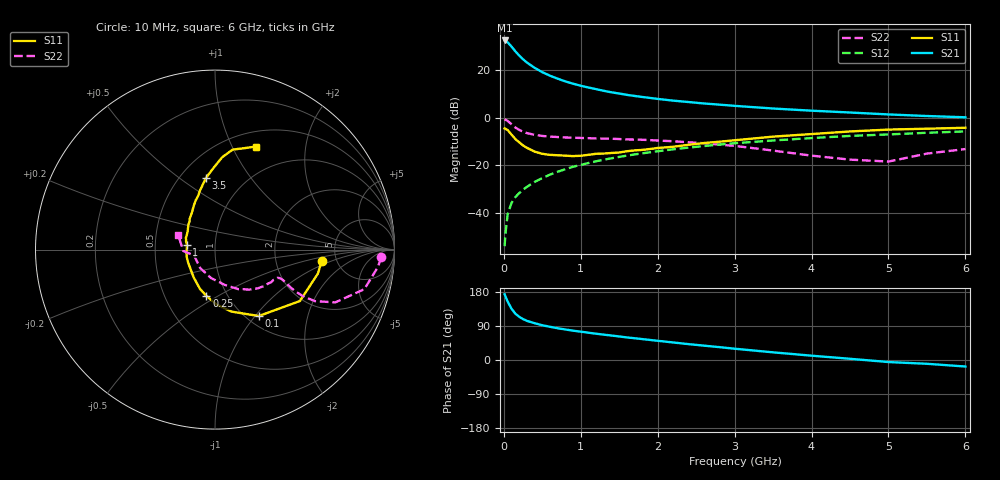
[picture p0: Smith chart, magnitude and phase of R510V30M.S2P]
! SIEMENS Small Signal Semiconductors
! BFR183
! Si NPN RF Bipolar Junction Transistor in SOT23
! VCE = 10 V  IC = 30 mA
! Common Emitter S-Parameters:  May  1996
# GHz  S  MA  R  50
!  f  S11  S21  S12  S22
! GHz  MAG  ANG  MAG  ANG  MAG  ANG  MAG  ANG
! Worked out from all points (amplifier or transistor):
!   36 points, 10 MHz to 6 GHz, reference 50 ohm
!   highest |S21| = 32.5 dB at 10 MHz (marker M1)
!   |S21| within 3 dB of that: start of sweep to 110.2 MHz
!   unconditionally stable (mu >= 1): 517 MHz to 2.553 GHz
!   at 250 MHz: K = 0.84, MSG = 27.4 dB, |S12| = -30.2 dB
!   at 1.4 GHz: K = 1.04, MAG = 12.6 dB, |S12| = -17.0 dB
!   at 6 GHz: K = 0.90, MSG = 3.0 dB, |S12| = -5.7 dB
!   S11 on the Smith chart (normalised r, x): 10 MHz: 3.80, -0.78; 100 MHz: 1.13, -1.04; 250 MHz: 0.80, -0.44; 1 GHz: 0.73, +0.04; 3.5 GHz: 0.66, +0.63; 6 GHz: 0.67, +1.24
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0.01  0.5977 -6.3  42.35 173.5  0.002 71.9  0.9278 -2.6
0.02  0.5887 -13.1  41.73 168.2  0.0035 79.3  0.9128 -6.1
0.05  0.5531 -31.2  38.66 154.0  0.0094 74.8  0.8612 -14.8
0.1  0.4432 -56.6  31.42 135.3  0.0163 69.5  0.7317 -23.7
0.15  0.3575 -75.1  24.99 122.2  0.0216 68.5  0.6257 -27.3
0.2  0.3053 -88.7  20.4 114.1  0.0261 69.3  0.5562 -27.9
0.25  0.262 -100.6  17.01 107.9  0.0309 69.6  0.5091 -27.5
0.3  0.2337 -111.2  14.55 103.3  0.0353 69.9  0.4771 -26.8
0.4  0.1945 -127.9  11.26 97.1  0.0449 71.5  0.4387 -25.2
0.5  0.1749 -140.8  9.117 91.7  0.0541 72.1  0.4157 -24.2
0.6  0.1664 -154.1  7.68 87.6  0.0639 72.2  0.4032 -23.8
0.7  0.1632 -164.3  6.649 83.8  0.0734 72.3  0.3941 -23.8
0.8  0.1602 -174.1  5.829 80.5  0.0831 71.2  0.3862 -24.1
1  0.1592 169.9  4.729 74.7  0.1022 70.2  0.3772 -25.2
1.1  0.1671 164.6  4.337 72.1  0.1121 69.5  0.3732 -26.5
1.3  0.1773 152.2  3.694 66.9  0.132 67.8  0.3649 -28.3
1.6  0.1985 138.7  3.039 59.6  0.1604 64.8  0.3515 -32.4
2.2  0.2458 121.2  2.3 46.3  0.2176 58.1  0.322 -42.1
3.5  0.4021 97.2  1.569 20.2  0.3338 41.8  0.2045 -74.4
4.5  0.5167 85.5  1.293 3.2  0.4166 29.4  0.132 -128.7
5.5  0.5905 73.4  1.091 -10.0  0.4848 18.3  0.1769 -177.6
6  0.6174 68.4  1.026 -17.2  0.5179 11.0  0.2204 158.4
